
FUNCTION_BLOCK FB51

TITLE = 'AFS_TEST'

//********************************************************************************
//
//
//
//********************************************************************************

//KNOW_HOW_PROTECT

VERSION: '1.0'
AUTHOR: MP
NAME: AFS_TEST
FAMILY: Std_Mdk

VAR_INPUT
INIT                :   BOOL            ;   // 1 = Initialisatie
AUTO                :   BOOL    :=TRUE  ;   // 1 = Testen automatisch
HAND                :   BOOL    :=FALSE ;   // 1 = Testen handmatig
UIT                 :   BOOL    :=FALSE ;   // 1 = Testen uitgeschakeld
HAND_START          :   BOOL    :=FALSE ;   // 1 = Testen handmatig gestart
DWA                 :   BOOL            ;   // 1 = DWA is actief
TEST_DAG            :   INT     := 4    ;   // Gewenste testdag (1 = Zondag)
CYCLUS              :   INT     := 1    ;   // Aantal weken tussen 2 testen
TIJD                :   TOD             ;   // Actuele tijd
DAG                 :   INT             ;   // Actuele dag ( 1=Zondag)
NIVEAU              :   REAL            ;   // Actueel niveau natte kelder
INSLAGPEIL          :   REAL            ;   // Inslagpeil
POMPEN              :   BOOL            ;   // 1 = 1 of meerdere pompen in bedrijf
AUTOMAAT            :   BOOL            ;   // 1 = Automaat bedrijf actief
AANTAL              :   INT     := 5    ;   // Aantal afsluiters voor test (max. 7)
AFSL1_OPEN          :   BOOL        ;   // 1 = openmelding
AFSL1_DICHT         :   BOOL        ;   // 1 = dichtmelding
AFSL1_ALARM         :   BOOL        ;   // 1 = alarm
AFSL2_OPEN          :   BOOL        ;   // 1 = openmelding
AFSL2_DICHT         :   BOOL        ;   // 1 = dichtmelding
AFSL2_ALARM         :   BOOL        ;   // 1 = alarm
AFSL3_OPEN          :   BOOL        ;   // 1 = openmelding
AFSL3_DICHT         :   BOOL        ;   // 1 = dichtmelding
AFSL3_ALARM         :   BOOL        ;   // 1 = alarm
AFSL4_OPEN          :   BOOL        ;   // 1 = openmelding
AFSL4_DICHT         :   BOOL        ;   // 1 = dichtmelding
AFSL4_ALARM         :   BOOL        ;   // 1 = alarm
AFSL5_OPEN          :   BOOL        ;   // 1 = openmelding
AFSL5_DICHT         :   BOOL        ;   // 1 = dichtmelding
AFSL5_ALARM         :   BOOL        ;   // 1 = alarm
AFSL6_OPEN          :   BOOL        ;   // 1 = openmelding
AFSL6_DICHT         :   BOOL        ;   // 1 = dichtmelding
AFSL6_ALARM         :   BOOL        ;   // 1 = alarm
AFSL7_OPEN          :   BOOL        ;   // 1 = openmelding
AFSL7_DICHT         :   BOOL        ;   // 1 = dichtmelding
AFSL7_ALARM         :   BOOL        ;   // 1 = alarm
RESET               :   BOOL        ;   // Reset puls.
END_VAR

VAR_IN_OUT
END_VAR

VAR_OUTPUT
TESTEN              :   BOOL        ;   // 1 = Testen is bezig
GETEST              :   BOOL        ;   // 1 = Vandaag getest
END_VAR

VAR_TEMP
END_VAR

VAR
STATUS              :   INT         ;   // Status van overblazen.
AFBREKEN            :   BOOL        ;   // 1 = Test wordt afgebroken.
ONDERBREKEN         :   BOOL        ;   // 1 = Test is onderbroken.
STORING             :   BOOL        ;   // 1 = Storing aan een klep
AUTO_START          :   BOOL        ;   // 1 = Voorwaarden autostart is aanwezig
TIJD_OK             :   BOOL        ;   // 1 = juiste tijd om te starten
DAG_OK              :   BOOL        ;   // 1 = juiste dag om te starten
NIVEAU_OK           :   BOOL        ;   // 1 = juiste niveau om te starten
HULP_MERKER         :   BOOL        ;   // Hulpmerker voor positieve flank afvangen
WEEK                :   INT         ;   // 0 = deze week testen
END_VAR

LABEL
END_LABEL

CONST
    TIJD1   := TOD#09:00:00.000;
    TIJD2   := TOD#15:00:00.000;
END_CONST


BEGIN
// Week naar 0 brengen. Elke zondag met 1 verlagen.
IF DAG = 1 AND NOT HULP_MERKER AND AUTO AND NOT (WEEK = 0) THEN
    WEEK := WEEK - 1;
    HULP_MERKER := TRUE;
END_IF;
IF DAG = 2 THEN
    HULP_MERKER := FALSE;
END_IF;

// Controleer of het tussen 09:00 uur en 15:00 uur is
IF (TIJD > TIJD1) AND (TIJD < TIJD2) THEN
    TIJD_OK := TRUE;
ELSE
    TIJD_OK := FALSE;
END_IF;

// Controleer of niveau lager is dan inslagpeil - 1.0%
IF (NIVEAU < (INSLAGPEIL - 1.0)) THEN
    NIVEAU_OK := TRUE;
ELSE
    NIVEAU_OK := FALSE;
END_IF;

// Als niveau te hoog dan onderbreken test.
IF NIVEAU >= INSLAGPEIL AND NOT HAND THEN
    ONDERBREKEN := TRUE;
END_IF;
IF ONDERBREKEN AND NIVEAU < (INSLAGPEIL - 1.0) AND NOT POMPEN OR UIT THEN
    ONDERBREKEN := FALSE;
END_IF;

// Controleer of vandaag testdag is.
IF DAG = TEST_DAG AND WEEK = 0 THEN
    DAG_OK := TRUE;
ELSE
    DAG_OK := FALSE;
END_IF;

// Als testdag geweest is de cyclus weer opnieuw Setten
IF DAG = (TEST_DAG + 1) AND WEEK <= 0 OR UIT THEN
    WEEK := CYCLUS;
    AFBREKEN := FALSE;
    GETEST := FALSE;
END_IF;

// Storing is als een klep alarm heeft.
IF AFSL1_ALARM OR AFSL2_ALARM OR AFSL3_ALARM OR AFSL4_ALARM OR AFSL5_ALARM OR AFSL6_ALARM OR AFSL7_ALARM THEN
    STORING := TRUE;
ELSE
    STORING := FALSE;
END_IF;

// Bepalen wanneer moet worden gestopt met testen.
IF STATUS <> 0 AND NOT HAND AND (NOT DWA OR NOT DAG_OK OR NOT TIJD_OK OR STORING OR NOT AUTOMAAT) THEN
    AFBREKEN := TRUE;
END_IF;

// Voorwaarden voor AUTO_START
IF DWA AND DAG_OK AND TIJD_OK AND NIVEAU_OK AND NOT POMPEN AND AUTOMAAT AND NOT STORING AND NOT GETEST THEN
    AUTO_START := TRUE;
ELSE
    AUTO_START := FALSE;
END_IF;

// Starten van testen.
IF STATUS = 0 AND (AANTAL >= 1) AND ((HAND AND HAND_START) OR (AUTO AND AUTO_START)) THEN
    TESTEN := TRUE;
    STATUS := 10;
END_IF;

IF STATUS = 10 AND AFSL1_DICHT THEN
    STATUS := 11;
END_IF;

IF STATUS = 11 AND AFSL1_OPEN THEN
    STATUS := 12;
END_IF;

IF STATUS = 12 AND NOT ONDERBREKEN AND (AANTAL > 1) THEN
    STATUS := 20;
ELSE
    IF STATUS = 12 AND NOT ONDERBREKEN AND (AANTAL = 1) THEN
        STATUS := 0;
        GETEST := TRUE;
    END_IF;
END_IF;

IF STATUS = 20 AND AFSL2_DICHT THEN
    STATUS := 21;
END_IF;

IF STATUS = 21 AND AFSL2_OPEN THEN
    STATUS := 22;
END_IF;

IF STATUS = 22 AND NOT ONDERBREKEN AND (AANTAL > 2) THEN
    STATUS := 30;
ELSE
    IF STATUS = 22 AND NOT ONDERBREKEN AND (AANTAL = 2) THEN
        STATUS := 0;
        GETEST := TRUE;
    END_IF;
END_IF;

IF STATUS = 30 AND AFSL3_DICHT THEN
    STATUS := 31;
END_IF;

IF STATUS = 31 AND AFSL3_OPEN THEN
    STATUS := 32;
END_IF;

IF STATUS = 32 AND NOT ONDERBREKEN AND (AANTAL > 3) THEN
    STATUS := 40;
ELSE
    IF STATUS = 32 AND NOT ONDERBREKEN AND (AANTAL = 3) THEN
        STATUS := 0;
        GETEST := TRUE;
    END_IF;
END_IF;

IF STATUS = 40 AND AFSL4_DICHT THEN
    STATUS := 41;
END_IF;

IF STATUS = 41 AND AFSL4_OPEN THEN
    STATUS := 42;
END_IF;

IF STATUS = 42 AND NOT ONDERBREKEN AND (AANTAL > 4) THEN
    STATUS := 50;
ELSE
    IF STATUS = 42 AND NOT ONDERBREKEN AND (AANTAL = 4) THEN
        STATUS := 0;
        GETEST := TRUE;
    END_IF;
END_IF;

IF STATUS = 50 AND AFSL5_DICHT THEN
    STATUS := 51;
END_IF;

IF STATUS = 51 AND AFSL5_OPEN THEN
    STATUS := 52;
END_IF;

IF STATUS = 52 AND NOT ONDERBREKEN AND (AANTAL > 5) THEN
    STATUS := 60;
ELSE
    IF STATUS = 52 AND NOT ONDERBREKEN AND (AANTAL = 5) THEN
        STATUS := 0;
        GETEST := TRUE;
    END_IF;
END_IF;

IF STATUS = 60 AND AFSL6_DICHT THEN
    STATUS := 61;
END_IF;

IF STATUS = 61 AND AFSL6_OPEN THEN
    STATUS := 62;
END_IF;

IF STATUS = 62 AND NOT ONDERBREKEN AND (AANTAL > 6) THEN
    STATUS := 70;
ELSE
    IF STATUS = 62 AND NOT ONDERBREKEN AND (AANTAL = 6) THEN
        STATUS := 0;
        GETEST := TRUE;
    END_IF;
END_IF;

IF STATUS = 70 AND AFSL7_DICHT THEN
    STATUS := 71;
END_IF;

IF STATUS = 71 AND AFSL7_OPEN THEN
    STATUS := 72;
END_IF;

IF STATUS = 72 THEN
    STATUS := 0;
    GETEST := TRUE;
END_IF;

// Wanneer wordt uitgeschakeld of wordt afgebroken, ga naar status 0.
IF (STATUS >= 10 AND STATUS <=72) AND (UIT OR AFBREKEN OR STORING) THEN
    STATUS := 0;
END_IF;



CASE STATUS OF
    10  :   TESTEN := TRUE;
    11  :   TESTEN := TRUE;
    12  :   TESTEN := TRUE;
    20  :   TESTEN := TRUE;
    21  :   TESTEN := TRUE;
    22  :   TESTEN := TRUE;
    30  :   TESTEN := TRUE;
    31  :   TESTEN := TRUE;
    32  :   TESTEN := TRUE;
    40  :   TESTEN := TRUE;
    41  :   TESTEN := TRUE;
    42  :   TESTEN := TRUE;
    50  :   TESTEN := TRUE;
    51  :   TESTEN := TRUE;
    52  :   TESTEN := TRUE;
    60  :   TESTEN := TRUE;
    61  :   TESTEN := TRUE;
    62  :   TESTEN := TRUE;
    70  :   TESTEN := TRUE;
    71  :   TESTEN := TRUE;
    72  :   TESTEN := TRUE;
    0   :   TESTEN := FALSE;
ELSE
    TESTEN := FALSE;
END_CASE;

END_FUNCTION_BLOCK
